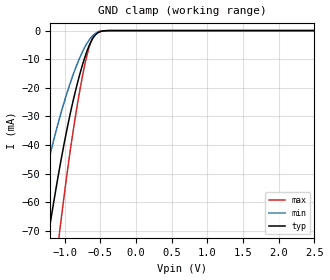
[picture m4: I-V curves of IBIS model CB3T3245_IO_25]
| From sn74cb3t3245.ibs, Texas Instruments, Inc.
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[Model]   CB3T3245_IO_25
Model_type  Terminator
| variable   typ   min   max
C_comp   3.98pF   3.29pF   4.36pF
| C_tri-state   3.98pF   3.29pF   4.36pF
[Temperature Range]   40   100   -40
| Ambient temperature   25   85   -40
[Voltage range]   2.5   2.3   2.7
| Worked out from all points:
|   GND clamp passes 1 mA (typ) near -0.55 V on its own axis
[GND Clamp]
| CB3T3245_IO_25
|   Voltage   I(typ)   I(min)   I(max)
-5V       -923.7mA   -700.9mA   -1.157A
-1.465V   -112.1mA   -73.18mA   -161.9mA
-1.42V    -104.1mA   -67.69mA   -150.7mA
-1.215V   -69.66mA   -44.66mA   -102.1mA
-1.075V   -48.84mA   -31.04mA   -71.64mA
-1.055V   -46.07mA   -29.25mA   -67.54mA
-895mV    -26.19mA   -16.48mA   -37.66mA
-750mV    -12.08mA   -7.489mA   -16.05mA
-650mV    -4.957mA   -3.097mA   -5.391mA
-545mV    -990.6uA   -722uA     -641.5uA
-345mV    -6.191uA   -9.353uA   -669.8nA
2.5V      223.5pA    2.228nA    50.35pA
